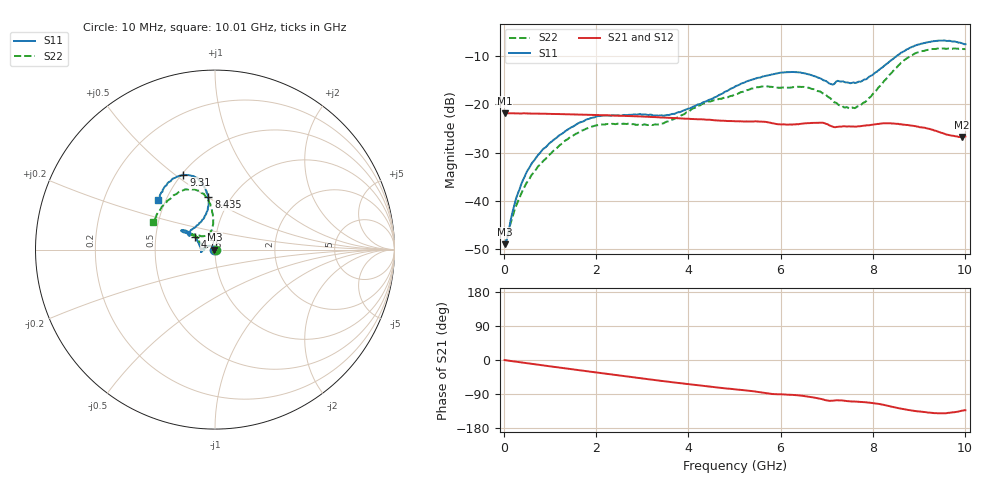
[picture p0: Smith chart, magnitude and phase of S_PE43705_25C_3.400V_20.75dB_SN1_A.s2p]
! Device ID: PE43705
! Serial: 1
! Insertion: A
! Impedance: 50 ohm
! Temp: 25C
! VDD: 3.400V
! Attenuation Step: 20.75dB
#  Hz  S  RI  R  50
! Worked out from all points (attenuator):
!   401 points, 10 MHz to 10.01 GHz, reference 50 ohm
!   highest |S21| = -21.80 dB at 10 MHz (marker M1); lowest = -26.8 dB at 9.935 GHz (marker M2)
!   lowest |S11| = -49.0 dB at 10 MHz (marker M3), VSWR 1.01, Z = 49.6 + j0.0391 ohm
!   |S11| at or under -10 dB: start of sweep to 8.516 GHz
!   |S22| runs from -49.4 to -8.4 dB; largest |S21 - S12| = 0.0012
!   S11 on the Smith chart (normalised r, x): 10 MHz: 0.99, +0.00; 4.76 GHz: 0.79, +0.11; 8.435 GHz: 0.79, +0.50; 9.31 GHz: 0.51, +0.53; 10.01 GHz: 0.46, +0.31
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1e7  -0.00353 0.000394  0.0812 -0.000324  0.0813 -0.000321  0.00338 0.000358
2.85e8  -0.00554 0.0101  0.0804 -0.00684  0.0804 -0.00679  0.00151 0.00939
5.6e8  -0.0132 0.0184  0.0793 -0.0133  0.0793 -0.0132  -0.00529 0.0165
1.01e9  -0.0344 0.0213  0.0762 -0.0233  0.0763 -0.0232  -0.0245 0.0187
1.685e9  -0.0654 0.00824  0.0692 -0.0366  0.0693 -0.0365  -0.0528 0.00879
2.185e9  -0.0764 -0.00732  0.0625 -0.0452  0.0626 -0.0452  -0.0618 -0.00131
3.36e9  -0.0761 -0.00634  0.0427 -0.0598  0.0428 -0.0596  -0.0617 0.00872
3.86e9  -0.0832 0.0181  0.0337 -0.063  0.0337 -0.063  -0.0727 0.0269
4.76e9  -0.1111 0.0707  0.0183 -0.0651  0.0185 -0.0651  -0.0967 0.0655
5.01e9  -0.127 0.0854  0.0146 -0.0653  0.0147 -0.0654  -0.1042 0.073
5.535e9  -0.1586 0.1031  0.00599 -0.0661  0.00612 -0.0662  -0.1218 0.0892
5.985e9  -0.1824 0.1093  -0.000572 -0.0621  -0.000242 -0.0619  -0.1194 0.0887
6.685e9  -0.175 0.0956  -0.00923 -0.0636  -0.0093 -0.0636  -0.12 0.0801
7.11e9  -0.1403 0.0805  -0.0178 -0.0563  -0.0179 -0.0565  -0.0818 0.0759
7.585e9  -0.1016 0.1346  -0.0196 -0.0557  -0.0194 -0.0554  -0.0372 0.084
7.885e9  -0.0607 0.1764  -0.023 -0.0563  -0.0225 -0.0565  -0.018 0.1116
8.36e9  -0.035 0.2752  -0.0334 -0.0543  -0.0334 -0.0542  -0.0136 0.2013
8.435e9  -0.0372 0.2926  -0.0353 -0.0527  -0.0355 -0.0529  -0.0169 0.2193
8.86e9  -0.0886 0.3862  -0.0414 -0.0438  -0.0408 -0.0441  -0.0763 0.3163
9.31e9  -0.176 0.4156  -0.0416 -0.0351  -0.0413 -0.0349  -0.1734 0.3321
9.935e9  -0.3078 0.3011  -0.0317 -0.0332  -0.0321 -0.033  -0.3287 0.1814
1.001e10  -0.3156 0.278  -0.0315 -0.0343  -0.0316 -0.0347  -0.3443 0.1522
